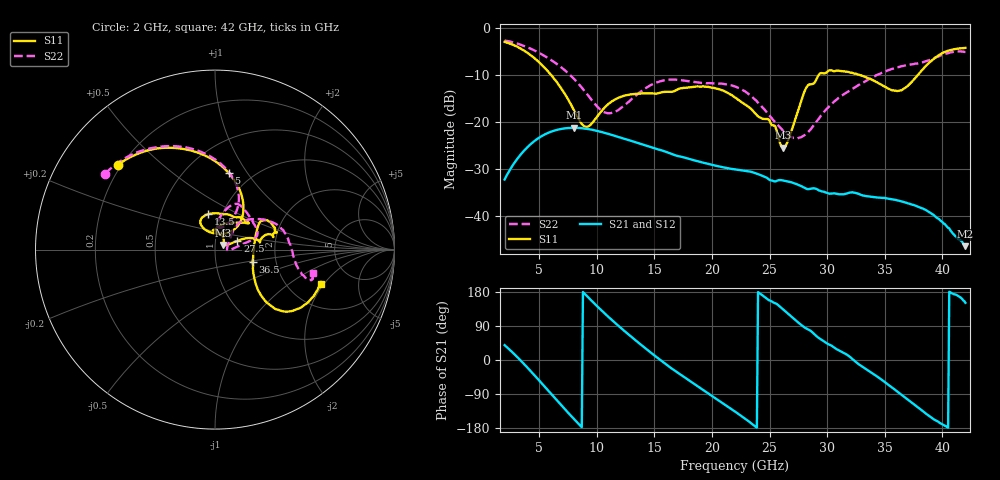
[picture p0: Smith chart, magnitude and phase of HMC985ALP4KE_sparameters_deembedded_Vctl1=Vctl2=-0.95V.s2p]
!s2p File: Measurements: S11, S21, S12, S22
# GHz S dB R 50.0
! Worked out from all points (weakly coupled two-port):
!   401 points, 2 GHz to 42 GHz, reference 50 ohm
!   highest |S21| = -21.23 dB at 8 GHz (marker M1); lowest = -46.5 dB at 42 GHz (marker M2)
!   lowest |S11| = -25.5 dB at 26.2 GHz (marker M3), VSWR 1.11, Z = 54.9 + j2.76 ohm
!   |S11| at or under -10 dB: 6.057 GHz to 29.25 GHz (23.2 GHz wide, 131 % of centre); 32.89 GHz to 37.85 GHz (4.963 GHz wide, 14 % of centre)
!   |S22| runs from -23.5 to -2.6 dB; largest |S21 - S12| = 0.00014
!   S11 on the Smith chart (normalised r, x): 2 GHz: 0.19, +0.36; 5 GHz: 0.78, +0.82; 13.5 GHz: 0.86, +0.35; 27.5 GHz: 1.28, +0.13; 36.5 GHz: 1.51, -0.21; 42 GHz: 3.00, -1.87
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2  -2.87 138.7  -32.28 39.1  -32.28 39.1  -2.57 145.3
3.4  -4.31 111.5  -26.94 -1.5  -26.94 -1.5  -3.49 122.6
5  -7.24 79.9  -23.34 -54.1  -23.34 -54.1  -5.22 97.8
6.3  -10.74 56.9  -21.84 -98.5  -21.85 -98.5  -7.18 79.7
8  -17.37 48.8  -21.23 -155.0  -21.24 -155.0  -10.71 63.1
8.7  -20.42 66.2  -21.32 -177.4  -21.32 -177.4  -12.65 60.5
9.4  -20.72 96.1  -21.56 160.9  -21.56 160.9  -14.81 61.6
11  -16.16 119.5  -22.53 114.1  -22.54 114.1  -18.13 78.1
13.5  -13.94 100.7  -24.43 48.6  -24.44 48.6  -14.12 79.6
15.4  -13.81 74.9  -25.91 3.0  -25.90 3.0  -11.37 68.4
18.9  -12.43 38.9  -28.47 -72.3  -28.47 -72.3  -11.57 41.2
22  -14.72 54.8  -30.10 -136.0  -30.10 -136.0  -12.41 17.0
24.9  -19.40 91.4  -32.16 158.7  -32.16 158.8  -18.33 7.1
26.2  -25.47 28.1  -32.51 132.5  -32.51 132.6  -21.91 -1.5
27.5  -17.45 21.2  -33.44 98.6  -33.45 98.7  -23.41 5.2
28.7  -11.89 9.6  -34.19 73.5  -34.18 73.5  -21.13 28.2
31  -9.02 20.4  -35.43 25.8  -35.43 25.8  -14.82 48.5
33.3  -10.36 31.8  -35.80 -22.4  -35.82 -22.3  -11.32 38.5
35.4  -12.96 10.7  -36.42 -67.5  -36.42 -67.5  -8.86 24.1
36.5  -13.17 -17.8  -37.01 -92.8  -37.02 -92.8  -8.04 15.5
39.6  -5.89 -42.5  -40.57 -162.2  -40.50 -162.3  -6.05 -15.3
42  -4.16 -18.1  -46.53 151.0  -46.67 150.5  -5.00 -13.6
